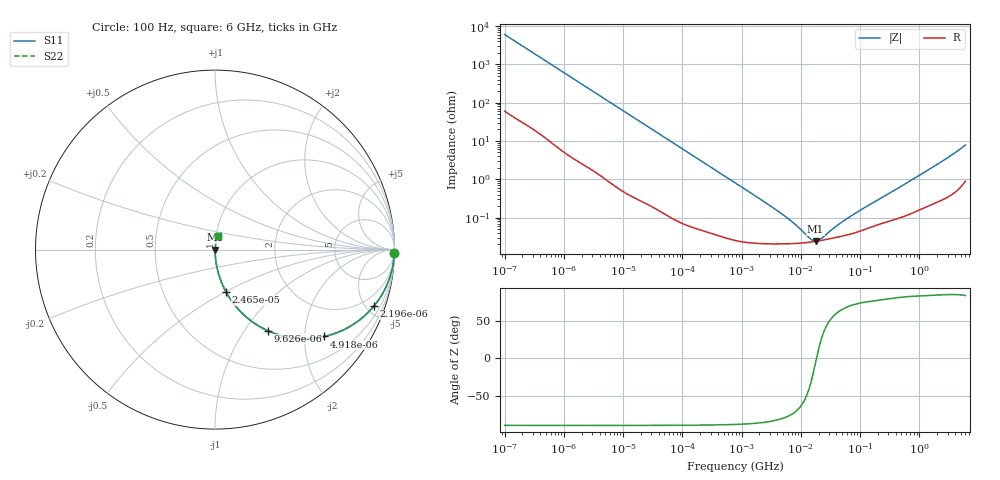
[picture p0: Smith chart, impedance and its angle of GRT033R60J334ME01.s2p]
!Murata Part Number: GRT033R60J334ME01
!These Parameters are Measured in Series Mode Connection
!Data Generated on Jun 19, 2026
!  o--ll--o
!Port1  Port2
!  o------o
!Operation Temp=25[degC], DC Bias Voltage=0[V]
!Freq. Start=100[Hz] Stop=6[GHz] 401[Steps]
# Hz S RI R 50
!Freq.(Hz) S11(Real) S11(Imag) S21(Real) S21(Imag) S12(Real) S12(Imag) S22(Real) S22(Imag)
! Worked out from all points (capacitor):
!   401 points, 100 Hz to 6 GHz, reference 50 ohm
!   read as one part in series: C = 264 nF near 109 Hz
!   lowest |Z| = 24.1 mohm at 17.79 MHz (marker M1)
!   series resonance near 18.42 MHz, so ESL is about 280 pH
!   S11 on the Smith chart (normalised r, x): 100 Hz: open; 2.196 kHz: 1.05, -5.57; 4.918 kHz: 1.02, -2.50; 9.626 kHz: 1.01, -1.28; 24.65 kHz: 1.00, -0.50; 6 GHz: 1.02, +0.16
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100  0.9996 -0.0166  0.000443 0.0166  0.000443 0.0166  0.9996 -0.0166
600  0.9895 -0.0974  0.0105 0.0974  0.0105 0.0974  0.9895 -0.0974
2008  0.9007 -0.2948  0.0993 0.2948  0.0993 0.2948  0.9007 -0.2948
2196  0.8839 -0.3162  0.1161 0.3162  0.1161 0.3162  0.8839 -0.3162
3287  0.7751 -0.4133  0.2249 0.4133  0.2249 0.4133  0.7751 -0.4133
4918  0.6091 -0.4839  0.3909 0.4839  0.3909 0.4839  0.6091 -0.4839
6728  0.4563 -0.4942  0.5437 0.4942  0.5437 0.4942  0.4563 -0.4942
9626  0.2925 -0.4511  0.7075 0.4511  0.7075 0.4511  0.2925 -0.4511
15062  0.1461 -0.3491  0.8539 0.3491  0.8539 0.3491  0.1461 -0.3491
24648  0.0613 -0.2354  0.9387 0.2354  0.9387 0.2354  0.0613 -0.2354
40335  0.0246 -0.15  0.9754 0.15  0.9754 0.15  0.0246 -0.15
129199  0.00293 -0.0482  0.9971 0.0482  0.9971 0.0482  0.00293 -0.0482
774597  0.00032 -0.00814  0.9997 0.00814  0.9997 0.00814  0.00032 -0.00814
5311619  0.000208 -0.00109  0.9998 0.00109  0.9998 0.00109  0.000208 -0.00109
1.555665e7  0.000232 -0.000112  0.9998 0.000112  0.9998 0.000112  0.000232 -0.000112
1.779312e7  0.00024 -2.24e-05  0.9998 2.24e-05  0.9998 2.24e-05  0.00024 -2.24e-05
2.128304e7  0.000251 9.41e-05  0.9997 -9.41e-05  0.9997 -9.41e-05  0.000251 9.41e-05
3.80911e7  0.0003 0.000486  0.9997 -0.000486  0.9997 -0.000486  0.0003 0.000486
6.817316e7  0.00037 0.001  0.9996 -0.001  0.9996 -0.001  0.00037 0.001
3.124326e8  0.000824 0.00422  0.9992 -0.00422  0.9992 -0.00422  0.000824 0.00422
2.048624e9  0.00316 0.0247  0.9968 -0.0247  0.9968 -0.0247  0.00316 0.0247
6e9  0.0147 0.0757  0.9853 -0.0757  0.9853 -0.0757  0.0147 0.0757
